| IBIS file stm32u3b5_3c5_lqfp144_smps.ibs
[IBIS ver] 4.2
[File name] stm32u3b5_3c5_lqfp144_smps.ibs
[File Rev] 0.1
[Date] 09-03-2026
[Source] Data Created at STMicroelectronics
[Notes]  File originated from ELDO simulations.
[Disclaimer]  This information is for modeling purpose only and is
   not guaranted. The information is subject to change without
   notice.
[Copyright] Copyright 2026 STMicroelectronics Inc.
|   Component stm32u3b5_3c5_lqfp144_smps
[Component] stm32u3b5_3c5_lqfp144_smps
[Manufacturer] STMicroelectronics
[Package]
| variable   typ   min   max
R_pkg  0  NA  NA
L_pkg  0  NA  NA
C_pkg  0  NA  NA
[Pin]   signal_name   model_name
1  PE2  io8_ft_100m
2  PE3  io8_ft_100m_hslv
3  PE4  io8_ft_100m
4  PE5  io8_ft_100m
5  PE6  io8_ft_100m
6  VBAT  power
7  PC13  io8_ft_100m_v33
8  PC14-OSC32_IN  io_ft_tamp
9  PC15-OSC32_OUT  io_ft_tamp
10  PF0  io8_ft_100m_hslv
11  PF1  io8_ft_100m_hslv
12  PF2  io8_ft_100m
13  PF3  io8_ft_100m
14  PF4  io8_ft_100m
15  PF5  io8_ft_100m
16  VSS  gnd
17  VDD  power
18  PF6  io8_ft_100m_hslv
19  PF7  io8_ft_100m_hslv
20  PF8  io8_ft_100m_hslv
21  PF9  io8_ft_100m_hslv
22  PF10  io8_ft_100m_hslv
23  PH0-OSC_IN  io8_ft_100m
24  PH1-OSC_OUT  io8_ft_100m
25  NRST  ioreset_v33
26  PC0  io8_ft_100m_hslv
27  PC1  io8_ft_100m_hslv
28  PC2  io8_ft_100m_hslv
29  PC3  io8_ft_100m_hslv
30  VSSA_VREFM  nc
31  VREFP  nc
32  VDDA  nc
33  PA0  io8_ft_100m
34  PA1  io8_ft_100m_hslv
35  PA2  io8_ft_100m_hslv
36  PA3  io8_ft_100m_hslv
37  VSS  gnd
38  VDD  power
39  PA4  io8_ft_100m_hslv
40  PA5  io8_ft_100m
41  PA6  io8_ft_100m_hslv
42  PA7  io8_ft_100m_hslv
43  PB0  io8_ft_100m_hslv
44  PB1  io8_ft_100m_hslv
45  PB2  io8_ft_100m_hslv
46  PF11  io8_ft_100m_hslv
47  PF12  io8_ft_100m
48  VSS  gnd
49  VDD  power
50  PF13  io8_ft_100m
51  PF14  io8_ft_100m_hslv
52  PF15  io8_ft_100m_hslv
53  PG0  io8_ft_100m
54  PG1  io8_ft_100m
55  PE7  io8_ft_100m
56  PE8  io8_ft_100m
57  PE9  io8_ft_100m_hslv
58  VSS  gnd
59  VDD  power
60  PE10  io8_ft_100m_hslv
61  PE11  io8_ft_100m_hslv
62  PE12  io8_ft_100m_hslv
63  PE13  io8_ft_100m_hslv
64  PE14  io8_ft_100m_hslv
65  PE15  io8_ft_100m_hslv
66  PB10  io8_ft_100m_hslv
67  PB11  io8_ft_100m_hslv
68  VLXSMPS  nc
69  VDDSMPS  nc
70  VSSSMPS  nc
71  VDD11  nc
72  VSS  gnd
73  VDD  power
74  PB13  io8_ft_100m_hslv
75  PB14  io8_ft_100m_hslv
76  PB15  io8_ft_100m
77  PD8  io8_ft_100m
78  PD9  io8_ft_100m
79  PD10  io8_ft_100m
80  PD11  io8_ft_100m_hslv
81  PD12  io8_ft_100m_hslv
82  PD13  io8_ft_100m_hslv
83  VSS  gnd
84  VDD  power
85  PD14  io8_ft_100m
86  PD15  io8_ft_100m
87  PG2  io8_ft_100m_hslv
88  PG3  io8_ft_100m_hslv
89  PG4  io8_ft_100m_hslv
90  PG5  io8_ft_100m_hslv
91  PG6  io8_ft_100m_hslv
92  PG7  io8_ft_100m_hslv
93  PG8  io8_ft_100m_hslv
94  VSS  gnd
95  VDDIO2  power
96  PC6  io8_ft_100m_hslv
97  PC7  io8_ft_100m_hslv
98  PC8  io8_ft_100m_hslv
99  PC9  io8_ft_100m_hslv
100  PA8  io8_ft_100m_hslv
101  PA9  io8_ft_100m
102  PA10  io8_ft_100m
103  PA11  io8usb_ft_phy
104  PA12  io8usb_ft_phy
105  PA13  io8_ft_100m
106  VDDUSB  power
107  VSS  gnd
108  VDD  power
109  PA14  io8_ft_100m
110  PA15  io8_ft_100m
111  PC10  io8_ft_100m_hslv
112  PC11  io8_ft_100m_hslv
113  PC12  io8_ft_100m_hslv
114  PD0  io8_ft_100m
115  PD1  io8_ft_100m
116  PD2  io8_ft_100m_hslv
117  PD3  io8_ft_100m_hslv
118  PD4  io8_ft_100m_hslv
119  PD5  io8_ft_100m_hslv
120  VSS  gnd
121  VDD  power
122  PD6  io8_ft_100m_hslv
123  PD7  io8_ft_100m_hslv
124  PG9  io8_ft_100m_hslv
125  PG10  io8_ft_100m_hslv
126  PG12  io8_ft_100m_hslv
127  PG13  io8_ft_100m_hslv
128  PG14  io8_ft_100m_hslv
129  VSS  gnd
130  VDDIO2  power
131  PG15  io8_ft_100m_hslv
132  PB3  io8_ft_100m_hslv
133  PB4  io8_ft_100m_hslv
134  PB5  io8_ft_100m_hslv
135  PB6  io8_ft_100m_hslv
136  PB7  io8_ft_100m_hslv
137  PH3-BOOT0  io8_ft_100m_hslv
138  PB8  io8_ft_100m_hslv
139  PB9  io8_ft_100m_hslv
140  PE0  io8_ft_100m
141  PE1  io8_ft_100m
142  VDD11  nc
143  VSS  gnd
144  VDD  power
[Package Model]   42a-lqfp-20x20-144-251212
[Pin Mapping]   pulldown_ref   pullup_ref   | Comment
1  gndio  vddio
2  gndio  vddio
3  gndio  vddio
4  gndio  vddio
5  gndio  vddio
6  nc  vsw
7  gndio  vsw
8  gndio  vsw
9  gndio  vsw
10  gndio  vddio
11  gndio  vddio
12  gndio  vddio
13  gndio  vddio
14  gndio  vddio
15  gndio  vddio
16  gndio  nc
17  nc  vddio
18  gndio  vddio
19  gndio  vddio
20  gndio  vddio
21  gndio  vddio
22  gndio  vddio
23  gndio  vddio
24  gndio  vddio
25  gndio  vddio
26  gndio  vddio
27  gndio  vddio
28  gndio  vddio
29  gndio  vddio
30  nc  nc
31  nc  nc
32  nc  nc
33  gndio  vddio
34  gndio  vddio
35  gndio  vddio
36  gndio  vddio
37  gndio  nc
38  nc  vddio
39  gndio  vddio
40  gndio  vddio
41  gndio  vddio
42  gndio  vddio
43  gndio  vddio
44  gndio  vddio
45  gndio  vddio
46  gndio  vddio
47  gndio  vddio
48  gndio  nc
49  nc  vddio
50  gndio  vddio
51  gndio  vddio
52  gndio  vddio
53  gndio  vddio
54  gndio  vddio
55  gndio  vddio
56  gndio  vddio
57  gndio  vddio
58  gndio  nc
59  nc  vddio
60  gndio  vddio
61  gndio  vddio
62  gndio  vddio
63  gndio  vddio
64  gndio  vddio
65  gndio  vddio
66  gndio  vddio
67  gndio  vddio
68  nc  nc
69  nc  nc
70  nc  nc
71  nc  nc
72  gndio  nc
73  nc  vddio
74  gndio  vddio
75  gndio  vddio
76  gndio  vddio
77  gndio  vddio
78  gndio  vddio
79  gndio  vddio
80  gndio  vddio
81  gndio  vddio
82  gndio  vddio
83  gndio  nc
84  nc  vddio
85  gndio  vddio
86  gndio  vddio
87  gndio  vddio2
88  gndio  vddio2
89  gndio  vddio2
90  gndio  vddio2
91  gndio  vddio2
92  gndio  vddio2
93  gndio  vddio2
94  gndio  nc
95  nc  vddio2
96  gndio  vddio
97  gndio  vddio
98  gndio  vddio
99  gndio  vddio
100  gndio  vddio
101  gndio  vddio
102  gndio  vddio
103  gndio  vddusb  | Depending on IO usage
| 103  gndio  vddio  | Depending on IO usage
104  gndio  vddusb  | Depending on IO usage
| 104  gndio  vddio  | Depending on IO usage
105  gndio  vddio
106  nc  vddusb
107  gndio  nc
108  nc  vddio
109  gndio  vddio
110  gndio  vddio
111  gndio  vddio
112  gndio  vddio
113  gndio  vddio
114  gndio  vddio
115  gndio  vddio
116  gndio  vddio
117  gndio  vddio
118  gndio  vddio
119  gndio  vddio
120  gndio  nc
121  nc  vddio
122  gndio  vddio
123  gndio  vddio
124  gndio  vddio2
125  gndio  vddio2
126  gndio  vddio2
127  gndio  vddio2
128  gndio  vddio2
129  gndio  nc
130  nc  vddio2
131  gndio  vddio2
132  gndio  vddio
133  gndio  vddio
134  gndio  vddio
135  gndio  vddio
136  gndio  vddio
137  gndio  vddio
138  gndio  vddio
139  gndio  vddio
140  gndio  vddio
141  gndio  vddio
142  nc  nc
143  gndio  nc
144  nc  vddio
|[Diff Pin]  inv_pin  vdiff  tdelay_typ  tdelay_min  tdelay_max
|104  103  NA  NA  NA  NA
[Model Selector] io8_ft_100m
io8_ft_100m_ls_1v2  "GPIO 100MHz - 5V tolerant - low speed - 1.2V range"
io8_ft_100m_ls_1v8  "GPIO 100MHz - 5V tolerant - low speed - 1.8V range"
io8_ft_100m_ls_3v3  "GPIO 100MHz - 5V tolerant - low speed - 3.3V range"
io8_ft_100m_ms_1v2  "GPIO 100MHz - 5V tolerant - med speed - 1.2V range"
io8_ft_100m_ms_1v8  "GPIO 100MHz - 5V tolerant - med speed - 1.8V range"
io8_ft_100m_ms_3v3  "GPIO 100MHz - 5V tolerant - med speed - 3.3V range"
io8_ft_100m_fs_1v2  "GPIO 100MHz - 5V tolerant - fast speed - 1.2V range"
io8_ft_100m_fs_1v8  "GPIO 100MHz - 5V tolerant - fast speed - 1.8V range"
io8_ft_100m_fs_3v3  "GPIO 100MHz - 5V tolerant - fast speed - 3.3V range"
io8_ft_100m_hs_1v2  "GPIO 100MHz - 5V tolerant - high speed - 1.2V range"
io8_ft_100m_hs_1v8  "GPIO 100MHz - 5V tolerant - high speed - 1.8V range"
io8_ft_100m_hs_3v3  "GPIO 100MHz - 5V tolerant - high speed - 3.3V range"
[Model Selector] io8_ft_100m_hslv
io8_ft_100m_ls_1v2  "GPIO 100MHz - 5V tolerant - low speed - 1.2V range"
io8_ft_100m_ls_1v8  "GPIO 100MHz - 5V tolerant - low speed - 1.8V range"
io8_ft_100m_ls_3v3  "GPIO 100MHz - 5V tolerant - low speed - 3.3V range"
io8_ft_100m_ms_1v2  "GPIO 100MHz - 5V tolerant - med speed - 1.2V range"
io8_ft_100m_ms_1v8  "GPIO 100MHz - 5V tolerant - med speed - 1.8V range"
io8_ft_100m_ms_3v3  "GPIO 100MHz - 5V tolerant - med speed - 3.3V range"
io8_ft_100m_fs_1v2  "GPIO 100MHz - 5V tolerant - fast speed - 1.2V range"
io8_ft_100m_fs_1v8  "GPIO 100MHz - 5V tolerant - fast speed - 1.8V range"
io8_ft_100m_fs_3v3  "GPIO 100MHz - 5V tolerant - fast speed - 3.3V range"
io8_ft_100m_hs_1v2  "GPIO 100MHz - 5V tolerant - high speed - 1.2V range"
io8_ft_100m_hs_1v8  "GPIO 100MHz - 5V tolerant - high speed - 1.8V range"
io8_ft_100m_hs_3v3  "GPIO 100MHz - 5V tolerant - high speed - 3.3V range"
io8_ft_100m_hslv_ls_1v2  "GPIO 100MHz low voltage optimization - 5V tolerant - low speed - 1.2V range"
io8_ft_100m_hslv_ls_1v8  "GPIO 100MHz low voltage optimization - 5V tolerant - low speed - 1.8V range"
io8_ft_100m_hslv_ls_2v5  "GPIO 100MHz low voltage optimization - 5V tolerant - low speed - 3.3V range"
io8_ft_100m_hslv_ms_1v2  "GPIO 100MHz low voltage optimization - 5V tolerant - med speed - 1.2V range"
io8_ft_100m_hslv_ms_1v8  "GPIO 100MHz low voltage optimization - 5V tolerant - med speed - 1.8V range"
io8_ft_100m_hslv_ms_2v5  "GPIO 100MHz low voltage optimization - 5V tolerant - med speed - 3.3V range"
io8_ft_100m_hslv_fs_1v2  "GPIO 100MHz low voltage optimization - 5V tolerant - fast speed - 1.2V range"
io8_ft_100m_hslv_fs_1v8  "GPIO 100MHz low voltage optimization - 5V tolerant - fast speed - 1.8V range"
io8_ft_100m_hslv_fs_2v5  "GPIO 100MHz low voltage optimization - 5V tolerant - fast speed - 3.3V range"
io8_ft_100m_hslv_hs_1v2  "GPIO 100MHz low voltage optimization - 5V tolerant - high speed - 1.2V range"
io8_ft_100m_hslv_hs_1v8  "GPIO 100MHz low voltage optimization - 5V tolerant - high speed - 1.8V range"
io8_ft_100m_hslv_hs_2v5  "GPIO 100MHz low voltage optimization - 5V tolerant - high speed - 3.3V range"
[Model Selector] io8_ft_100m_v33
io8_ft_100m_v33_ls_1v2  "GPIO_V33 100MHz - 5V tolerant - low speed - 1.2V range"
io8_ft_100m_v33_ls_1v8  "GPIO_V33 100MHz - 5V tolerant - low speed - 1.8V range"
io8_ft_100m_v33_ls_3v3  "GPIO_V33 100MHz - 5V tolerant - low speed - 3.3V range"
io8_ft_100m_v33_ms_1v2  "GPIO_V33 100MHz - 5V tolerant - med speed - 1.2V range"
io8_ft_100m_v33_ms_1v8  "GPIO_V33 100MHz - 5V tolerant - med speed - 1.8V range"
io8_ft_100m_v33_ms_3v3  "GPIO_V33 100MHz - 5V tolerant - med speed - 3.3V range"
io8_ft_100m_v33_fs_1v2  "GPIO_V33 100MHz - 5V tolerant - fast speed - 1.2V range"
io8_ft_100m_v33_fs_1v8  "GPIO_V33 100MHz - 5V tolerant - fast speed - 1.8V range"
io8_ft_100m_v33_fs_3v3  "GPIO_V33 100MHz - 5V tolerant - fast speed - 3.3V range"
io8_ft_100m_v33_hs_1v2  "GPIO_V33 100MHz - 5V tolerant - high speed - 1.2V range"
io8_ft_100m_v33_hs_1v8  "GPIO_V33 100MHz - 5V tolerant - high speed - 1.8V range"
io8_ft_100m_v33_hs_3v3  "GPIO_V33 100MHz - 5V tolerant - high speed - 3.3V range"
[Model Selector] io8usb_ft_phy
io8_ft_100m_ls_1v2  "GPIO 100MHz - 5V tolerant - low speed - 1.2V range"
io8_ft_100m_ls_1v8  "GPIO 100MHz - 5V tolerant - low speed - 1.8V range"
io8_ft_100m_ls_3v3  "GPIO 100MHz - 5V tolerant - low speed - 3.3V range"
io8_ft_100m_ms_1v2  "GPIO 100MHz - 5V tolerant - med speed - 1.2V range"
io8_ft_100m_ms_1v8  "GPIO 100MHz - 5V tolerant - med speed - 1.8V range"
io8_ft_100m_ms_3v3  "GPIO 100MHz - 5V tolerant - med speed - 3.3V range"
io8_ft_100m_fs_1v2  "GPIO 100MHz - 5V tolerant - fast speed - 1.2V range"
io8_ft_100m_fs_1v8  "GPIO 100MHz - 5V tolerant - fast speed - 1.8V range"
io8_ft_100m_fs_3v3  "GPIO 100MHz - 5V tolerant - fast speed - 3.3V range"
io8_ft_100m_hs_1v2  "GPIO 100MHz - 5V tolerant - high speed - 1.2V range"
io8_ft_100m_hs_1v8  "GPIO 100MHz - 5V tolerant - high speed - 1.8V range"
io8_ft_100m_hs_3v3  "GPIO 100MHz - 5V tolerant - high speed - 3.3V range"
io8usb_ft_phy_hs_3v3   "USB full speed"
io8usb_ft_phy_ls_3v3   "USB low speed"
[Model Selector] io_ft_tamp
io_ft_tamp_ls_1v2 "io8_ft tamp low speed @ 1.2V"
io_ft_tamp_ls_1v8 "io8_ft tamp low speed @ 1.8V"
io_ft_tamp_ls_3v3 "io8_ft tamp low speed @ 3.3V"
io_ft_tamp_ms_1v2 "io8_ft tamp med speed @ 1.2V"
io_ft_tamp_ms_1v8 "io8_ft tamp med speed @ 1.8V"
io_ft_tamp_ms_3v3 "io8_ft tamp med speed @ 3.3V"
io_ft_tamp_fs_1v2 "io8_ft tamp fast speed @ 1.2V"
io_ft_tamp_fs_1v8 "io8_ft tamp fast speed @ 1.8V"
io_ft_tamp_fs_3v3 "io8_ft tamp fast speed @ 3.3V"
io_ft_tamp_hs_1v2 "io8_ft tamp high speed @ 1.2V"
io_ft_tamp_hs_1v8 "io8_ft tamp high speed @ 1.8V"
io_ft_tamp_hs_3v3 "io8_ft tamp high speed @ 3.3V"
[Model Selector] ioreset_v33
ioreset_v33_1v2 "Reset PAD. 5V tolerant. 1.2V range"
ioreset_v33_1v8 "Reset PAD. 5V tolerant. 1.8V range"
ioreset_v33_3v3 "Reset PAD. 5V tolerant. 3.3V range"
[Define Package Model]  42a-lqfp-20x20-144-251212
[Manufacturer]  Unknown
[OEM]  Unknown
[Description]  None
[Number Of Pins]  138
[Pin Numbers]
| Pin Num   Terminal Name
25 | NRST
33 | PA0
34 | PA1
35 | PA2
36 | PA3
39 | PA4
40 | PA5
41 | PA6
42 | PA7
100 | PA8
101 | PA9
102 | PA10
103 | PA11
104 | PA12
105 | PA13
109 | PA14
110 | PA15
43 | PB0
44 | PB1
45 | PB2
132 | PB3
133 | PB4
134 | PB5
135 | PB6
136 | PB7
138 | PB8
139 | PB9
66 | PB10
67 | PB11
74 | PB13
75 | PB14
76 | PB15
26 | PC0
27 | PC1
28 | PC2
29 | PC3
96 | PC6
97 | PC7
98 | PC8
99 | PC9
111 | PC10
112 | PC11
113 | PC12
7 | PC13
8 | PC14-OSC32_IN
9 | PC15-OSC32_OUT
114 | PD0
115 | PD1
116 | PD2
117 | PD3
118 | PD4
119 | PD5
122 | PD6
123 | PD7
77 | PD8
78 | PD9
79 | PD10
80 | PD11
81 | PD12
82 | PD13
85 | PD14
86 | PD15
140 | PE0
141 | PE1
1 | PE2
2 | PE3
3 | PE4
4 | PE5
5 | PE6
55 | PE7
56 | PE8
57 | PE9
60 | PE10
61 | PE11
62 | PE12
63 | PE13
64 | PE14
65 | PE15
10 | PF0
11 | PF1
12 | PF2
13 | PF3
14 | PF4
15 | PF5
18 | PF6
19 | PF7
20 | PF8
21 | PF9
22 | PF10
46 | PF11
47 | PF12
50 | PF13
51 | PF14
52 | PF15
53 | PG0
54 | PG1
87 | PG2
88 | PG3
89 | PG4
90 | PG5
91 | PG6
92 | PG7
93 | PG8
124 | PG9
125 | PG10
126 | PG12
127 | PG13
128 | PG14
131 | PG15
23 | PH0-OSC_IN
24 | PH1-OSC_OUT
137 | PH3-BOOT0
71 | VDD11
142 | VDD11
6 | VBAT
17 | VDD
38 | VDD
49 | VDD
59 | VDD
73 | VDD
84 | VDD
108 | VDD
121 | VDD
144 | VDD
32 | VDDA
95 | VDDIO2
130 | VDDIO2
69 | VDDSMPS
106 | VDDUSB
68 | VLXSMPS
31 | VREFP
16 | VSS
83 | VSS
94 | VSS
120 | VSS
129 | VSS
30 | VSSA_VREFM
70 | VSSSMPS
|[Merged Pins]  16
|37  |  VSS
|48  |  VSS
|58  |  VSS
|72  |  VSS
|107  |  VSS
|143  |  VSS
[Model Data]
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[End Model Data]
[End Package Model]
|End [Component]
| Models and submodels in the file (53): io8_ft_100m_fs_1v2 (I/O), io8_ft_100m_fs_1v8 (I/O), io8_ft_100m_fs_3v3 (I/O), io8_ft_100m_hs_1v2 (I/O), io8_ft_100m_hs_1v8 (I/O), io8_ft_100m_hs_3v3 (I/O), io8_ft_100m_hslv_fs_1v2 (I/O), io8_ft_100m_hslv_fs_1v8 (I/O), io8_ft_100m_hslv_fs_2v5 (I/O), io8_ft_100m_hslv_hs_1v2 (I/O), io8_ft_100m_hslv_hs_1v8 (I/O), io8_ft_100m_hslv_hs_2v5 (I/O), io8_ft_100m_hslv_ls_1v2 (I/O), io8_ft_100m_hslv_ls_1v8 (I/O), io8_ft_100m_hslv_ls_2v5 (I/O), io8_ft_100m_hslv_ms_1v2 (I/O), io8_ft_100m_hslv_ms_1v8 (I/O), io8_ft_100m_hslv_ms_2v5 (I/O), io8_ft_100m_ls_1v2 (I/O), io8_ft_100m_ls_1v8 (I/O), io8_ft_100m_ls_3v3 (I/O), io8_ft_100m_ms_1v2 (I/O), io8_ft_100m_ms_1v8 (I/O), io8_ft_100m_ms_3v3 (I/O), io8_ft_100m_v33_fs_1v2 (I/O), io8_ft_100m_v33_fs_1v8 (I/O), io8_ft_100m_v33_fs_3v3 (I/O), io8_ft_100m_v33_hs_1v2 (I/O), io8_ft_100m_v33_hs_1v8 (I/O), io8_ft_100m_v33_hs_3v3 (I/O), io8_ft_100m_v33_ls_1v2 (I/O), io8_ft_100m_v33_ls_1v8 (I/O), io8_ft_100m_v33_ls_3v3 (I/O), io8_ft_100m_v33_ms_1v2 (I/O), io8_ft_100m_v33_ms_1v8 (I/O), io8_ft_100m_v33_ms_3v3 (I/O), io8usb_ft_phy_hs_3v3 (I/O), io8usb_ft_phy_ls_3v3 (I/O), io_ft_tamp_fs_1v2 (I/O), io_ft_tamp_fs_1v8 (I/O), io_ft_tamp_fs_3v3 (I/O), io_ft_tamp_hs_1v2 (I/O), io_ft_tamp_hs_1v8 (I/O), io_ft_tamp_hs_3v3 (I/O), io_ft_tamp_ls_1v2 (I/O), io_ft_tamp_ls_1v8 (I/O), io_ft_tamp_ls_3v3 (I/O), io_ft_tamp_ms_1v2 (I/O), io_ft_tamp_ms_1v8 (I/O), io_ft_tamp_ms_3v3 (I/O), ioreset_v33_1v2 (I/O_open_drain), ioreset_v33_1v8 (I/O_open_drain), ioreset_v33_3v3 (I/O_open_drain)
